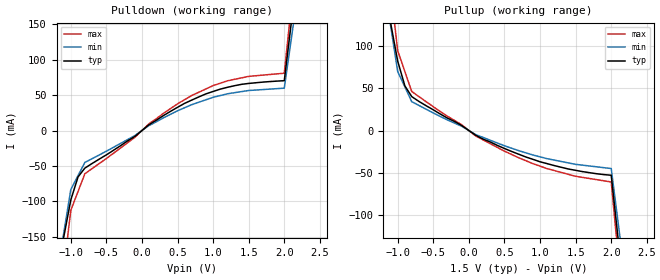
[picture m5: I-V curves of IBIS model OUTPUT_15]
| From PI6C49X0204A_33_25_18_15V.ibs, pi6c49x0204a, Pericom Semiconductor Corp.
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|   Model OUTPUT_15
[Model] OUTPUT_15
Model_type Output
Vref = 0.0000V
Rref = 50ohms
Vmeas = 0.750V
| variable   typ   min   max
C_comp   2.000pF   1.8pF	2.2pF
[Voltage Range]   1.5   1.425  1.575
[POWER Clamp Reference]   1.500V   NA   NA
[GND Clamp Reference]   0.000V   0	 0
[Pullup Reference]   1.5   1.425   1.575
[Pulldown Reference]   0.000V   NA   NA
[Temperature Range]   25.00   85.00   -45.000
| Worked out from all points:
|   slope of the pulldown table from 0 to 0.225 V, typ, clamps not added: 14.1 ohm
|   slope of the pullup table from 0 to 0.225 V, typ, clamps not added: 20.5 ohm
[Pulldown]
| Voltage   I(typ)   I(min)  I(max)
-1.501V   -461.9mA   -392.6mA   -531.2mA
-1.1V     -151.1mA   NA         NA
-999.3mV  -97.83mA   -83.16mA   -112.5mA
-898.2mV  -65.44mA   NA         NA
-802mV    -52.94mA   -45mA      -60.88mA
-99.45mV  -8.35mA    -7.097mA   -9.602mA
99.45mV   8.25mA     7.012mA    9.487mA
700.9mV   42.95mA    36.51mA    49.39mA
1.202V    60.91mA    51.77mA    70.05mA
1.5V      66.36mA    56.41mA    76.31mA
2V        70.22mA    59.69mA    80.75mA
2.599V    566.4mA    481.4mA    651.3mA
[Pullup]   |Note: Vtable = Vcc - Voutput
| Voltage   I(typ)   I(min)   I(max)
-1.5V     403.8mA    343.2mA    464.4mA
-1.1V     128.3mA    NA         NA
-999.4mV  82.22mA    69.89mA    94.55mA
-898.2mV  52.83mA    NA         NA
-802mV    40.18mA    34.15mA    46.21mA
-99.45mV  5.88mA     4.998mA    6.762mA
99.44mV   -5.76mA    -4.896mA   -6.624mA
700.9mV   -28.06mA   -23.85mA   -32.27mA
1.1V      -39.25mA   -33.36mA   -45.14mA
1.5V      -47.14mA   -40.07mA   -54.21mA
2V        -52.97mA   -45.02mA   -60.92mA
2.597V    -517.9mA   -440.2mA   -595.6mA
[Ramp]
| variable   typ   min   max
dV/dt_r   1.5V/941.0p   1.5V/1041.0p   1.5V/841.0p
dV/dt_f   1.5V/806.0p   1.5V/1006.0p   1.5V/706.0p
R_load = 50ohms
